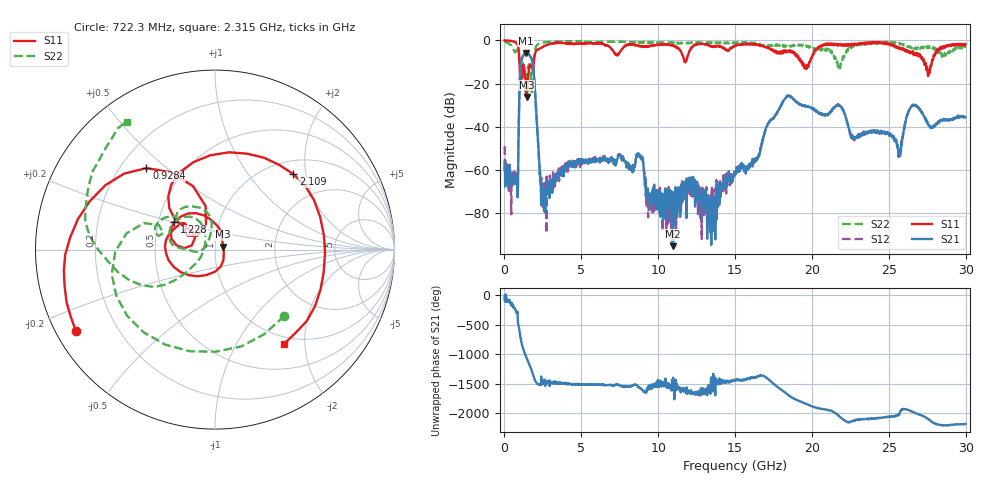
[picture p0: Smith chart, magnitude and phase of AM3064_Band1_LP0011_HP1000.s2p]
# Hz S DB R 50.0
!freq dBS11 angS11 dBS21 angS21 dBS12 angS12 dBS22 angS22
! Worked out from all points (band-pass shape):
!   1600 points, 10 MHz to 29.98 GHz, reference 50 ohm
!   highest |S21| = -5.78 dB at 1.397 GHz (marker M1); lowest = -95.2 dB at 10.98 GHz (marker M2)
!   |S21| within 3 dB of the highest: 1.124 GHz to 1.773 GHz (649.7 MHz wide, 44.9 % of centre)
!   lowest |S11| = -26.2 dB at 1.453 GHz (marker M3), VSWR 1.10, Z = 54.8 + j1.7 ohm
!   |S11| at or under -10 dB: 973.5 MHz to 1.913 GHz (939.7 MHz wide, 65.1 % of centre); 19.35 GHz to 19.83 GHz (475.9 MHz wide, 2.43 % of centre); 27.3 GHz to 27.79 GHz (494.9 MHz wide, 1.8 % of centre)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
!   |S22| runs from -25.1 to -0.3 dB; largest |S21 - S12| = 0.0061
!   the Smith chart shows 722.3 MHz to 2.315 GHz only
!   S11 on the Smith chart (normalised r, x): 722.3 MHz: 0.06, -0.27; 928.4 MHz: 0.31, +0.43; 1.228 GHz: 0.60, +0.20; 2.109 GHz: 1.28, +1.70; 2.315 GHz: 0.89, -1.61
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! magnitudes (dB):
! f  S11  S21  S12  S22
! 10 MHz  0.0  -59.7  -49.0  -0.3
! 722.3 MHz  -0.9  -63.5  -66.5  -5.4
! 928.4 MHz  -4.5  -39.8  -39.5  -6.0
! 1.228 GHz  -11.2  -7.1  -7.0  -11.3
! 1.397 GHz  -19.1  -5.8  -5.8  -21.4
! 1.453 GHz  -26.2  -5.8  -5.8  -16.6
! 1.828 GHz  -13.4  -10.3  -10.3  -17.6
! 2.109 GHz  -4.3  -38.2  -38.2  -2.3
! 2.315 GHz  -3.7  -60.9  -62.5  -1.3
! 2.54 GHz  -2.8  -70.6  -71.4  -0.9
! 5.015 GHz  -1.4  -56.0  -55.1  -0.7
! 8.745 GHz  -2.6  -53.4  -53.3  -1.1
! 9.363 GHz  -2.8  -70.5  -79.7  -1.0
! 10 GHz  -2.0  -74.5  -78.6  -0.9
! 10.98 GHz  -2.6  -95.2  -73.2  -1.0
! 13.6 GHz  -2.8  -79.5  -77.5  -1.2
! 15 GHz  -2.6  -62.3  -61.9  -1.3
! 18.36 GHz  -5.3  -26.0  -26.1  -3.0
! 19.99 GHz  -8.1  -31.4  -31.3  -3.4
! 25 GHz  -1.3  -43.4  -43.1  -1.1
! 27.56 GHz  -16.5  -38.8  -38.9  -2.9
! 29.98 GHz  -1.7  -35.5  -35.5  -3.3
